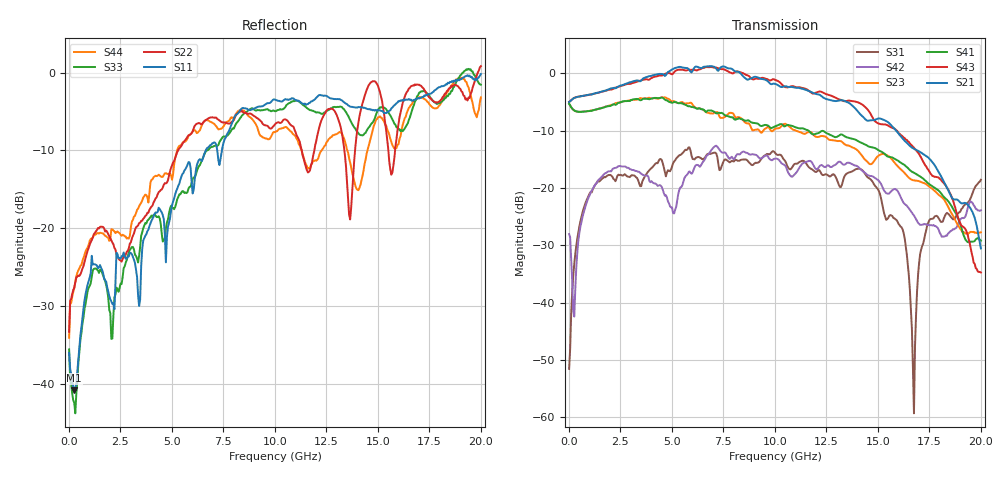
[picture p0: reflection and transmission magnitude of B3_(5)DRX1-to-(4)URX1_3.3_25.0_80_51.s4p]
!Agilent Technologies,N5225A,MY51451112,A.09.50.13
!Agilent N5225A: A.09.50.13
!Date: Sunday, March 12, 2017 05:21:13
!Correction: S11(Full 4 Port(1,2,3,4))
!S12(Full 4 Port(1,2,3,4))
!S13(Full 4 Port(1,2,3,4))
!S14(Full 4 Port(1,2,3,4))
!S21(Full 4 Port(1,2,3,4))
!S22(Full 4 Port(1,2,3,4))
!S23(Full 4 Port(1,2,3,4))
!S24(Full 4 Port(1,2,3,4))
!S31(Full 4 Port(1,2,3,4))
!S32(Full 4 Port(1,2,3,4))
!S33(Full 4 Port(1,2,3,4))
!S34(Full 4 Port(1,2,3,4))
!S41(Full 4 Port(1,2,3,4))
!S42(Full 4 Port(1,2,3,4))
!S43(Full 4 Port(1,2,3,4))
!S44(Full 4 Port(1,2,3,4))
!S4P File: Measurements: <S11,S12,S13,S14>,
!<S21,S22,S23,S24>,
!<S31,S32,S33,S34>,
!<S41,S42,S43,S44>:
# Hz S  dB  R 50
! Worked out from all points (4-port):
!   401 points, 10 MHz to 20 GHz, reference 50 ohm
!   strongest paths, dB at 10 MHz, 5.008 GHz, 10.01 GHz, 15 GHz, 20 GHz:
!     S21: -5.0, 0.7, -1.8, -7.9, -30.6
!     S43: -5.0, -0.2, -1.1, -8.7, -34.8
!     S41: -5.3, -5.1, -9.3, -13.4, -29.2
!     S23: -5.3, -4.9, -9.7, -14.4, -27.7
!     S42: -28.1, -23.4, -14.9, -18.6, -23.9
!     S31: -51.6, -16.3, -13.9, -20.2, -18.6
!   lowest |S11| = -40.8 dB at 259.9 MHz (marker M1), VSWR 1.02, Z = 50.3 - j0.872 ohm
!   |S11| at or under -10 dB: start of sweep to 6.642 GHz; 7.201 GHz to 7.427 GHz (225.5 MHz wide, 3.08 % of centre)
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1e7  -36.03 -39.0  -69.74 151.2  -52.91 22.7  -63.98 136.9
     -5.01 1.4  -33.30 39.2  -5.33 -180.0  -27.96 37.7
     -51.58 19.5  -65.86 126.9  -35.57 -45.4  -69.99 122.5
     -5.33 180.0  -28.06 38.1  -5.00 1.5  -34.09 45.2
2.59875e8  -40.84 -72.8  -49.70 53.4  -33.16 94.7  -50.38 52.9
           -4.30 -4.4  -27.64 -131.6  -6.48 166.8  -41.91 -161.4
           -33.24 95.5  -49.81 56.1  -42.45 -79.0  -50.58 53.9
           -6.48 165.9  -42.45 -171.6  -4.29 -5.2  -27.70 -137.7
5.2074e9  -15.22 86.0  -35.93 11.0  -15.05 29.9  -37.51 -4.7
          0.98 173.6  -10.62 142.4  -5.08 -31.6  -23.68 65.2
          -14.88 27.8  -36.33 8.4  -16.82 103.0  -42.77 -21.9
          -5.06 -47.9  -23.30 65.2  0.50 163.6  -10.50 120.5
8.30585e9  -4.84 37.5  -39.53 -99.5  -15.31 -1.4  -36.58 -139.7
           0.09 22.0  -4.97 79.6  -7.72 -156.7  -13.83 47.0
           -15.20 -1.9  -32.61 -124.0  -5.86 57.5  -32.06 -161.7
           -7.92 -179.8  -14.13 50.5  0.19 9.4  -4.81 44.9
1.22039e10  -2.86 -18.9  -33.95 -155.9  -16.86 -23.3  -35.39 164.2
            -3.82 -142.1  -6.54 68.3  -10.98 47.4  -15.91 38.9
            -17.17 -22.3  -34.17 -145.3  -5.20 -6.1  -33.09 170.3
            -10.22 10.2  -16.09 41.7  -3.18 -167.1  -10.23 -6.8
1.675162e10  -3.50 -76.7  -35.11 113.5  -53.36 -30.1  -36.51 85.4
             -13.15 19.7  -1.68 67.9  -18.69 178.0  -24.93 60.3
             -59.33 -113.1  -33.13 123.0  -4.13 -82.5  -33.37 82.9
             -17.36 126.3  -24.79 60.5  -12.97 -31.3  -3.69 -60.7
2e10  -0.18 -114.1  -33.00 63.0  -18.63 121.6  -35.47 21.4
      -30.56 -129.4  0.84 17.1  -27.74 41.3  -23.89 102.0
      -18.58 121.6  -33.98 40.1  -1.54 -87.6  -35.21 -7.6
      -29.20 -0.9  -23.90 102.8  -34.76 -154.8  -3.18 -136.5
